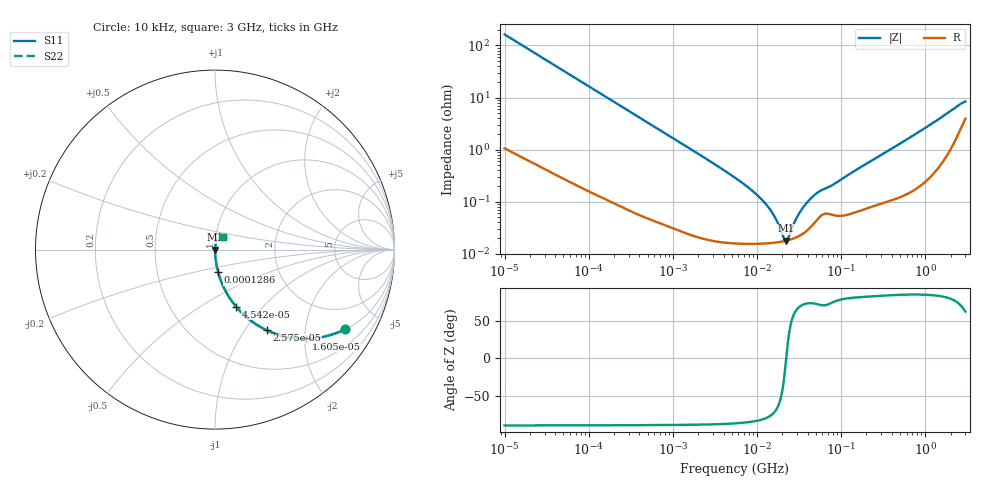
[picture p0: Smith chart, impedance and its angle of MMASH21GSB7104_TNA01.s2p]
! MMASH21GSB7104_TNA01  S-PARAMETER MODEL  ( Standard Model )
! Model Generated by TAIYO YUDEN Corporation (http://www.ty-top.com)
! Version 1.0
! TAIYO YUDEN Control No. 220601
! Copyright(c) 2013 TAIYO YUDEN CO.,LTD. All Rights Reserved.
! Product Description (link to TY-COMPAS)
! https://ds.yuden.co.jp/TYCOMPAS/or/detail?pn=MMASH21GSB7104KTNA01&u=M
! Products Name : Multilayer Ceramic Capacitors
! Characteristics :
!  Capacitance : 0.1 [uF] , Rated Voltage : 100 [V] , TCC : X7R
!  Case Size : 2.0 x 1.25 / 0.079 x 0.049 [mm/inch] , Thickness : 1.25 / 0.049 [mm/inch]
!  (Conditions: Temperature = 25 [degC] , DC Bias Voltage = 0 [V])
! External Node Assignments :
!  1  o---| |---o  2
! GND o---------o GND
! Frequency Range : 10kHz  -  3GHz  [ 401 STEP ]
# MHZ S RI R 50
! Freq[MHz].  S11 Real  S11 Imag  S21 Real  S21 Imag  S12 Real  S12 Imag  S22 Real  S22 Imag
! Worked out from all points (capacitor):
!   401 points, 10 kHz to 3 GHz, reference 50 ohm
!   read as one part in series: C = 97.7 nF near 10.65 kHz
!   lowest |Z| = 17.9 mohm at 21.93 MHz (marker M1)
!   series resonance near 22.24 MHz, so ESL is about 520 pH
!   S11 on the Smith chart (normalised r, x): 10 kHz: 1.02, -3.26; 16.05 kHz: 1.01, -2.03; 25.75 kHz: 1.01, -1.27; 45.42 kHz: 1.01, -0.72; 128.6 kHz: 1.00, -0.26; 3 GHz: 1.08, +0.15
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0.01  0.7247 -0.4434  0.2753 0.4434  0.2753 0.4434  0.7247 -0.4434
0.016047  0.5081 -0.4964  0.4919 0.4964  0.4919 0.4964  0.5081 -0.4964
0.02575  0.2886 -0.4494  0.7114 0.4494  0.7114 0.4494  0.2886 -0.4494
0.045421  0.1172 -0.3176  0.8828 0.3176  0.8828 0.3176  0.1172 -0.3176
0.082683  0.0397 -0.1906  0.9603 0.1906  0.9603 0.1906  0.0397 -0.1906
0.128563  0.0174 -0.1258  0.9826 0.1258  0.9826 0.1258  0.0174 -0.1258
0.683653  0.000984 -0.0243  0.999 0.0243  0.999 0.0243  0.000984 -0.0243
5.477226  0.000166 -0.00289  0.9998 0.00289  0.9998 0.00289  0.000166 -0.00289
9.070798  0.000157 -0.00155  0.9998 0.00155  0.9998 0.00155  0.000157 -0.00155
12.83117  0.000159 -0.000877  0.9998 0.000877  0.9998 0.000877  0.000159 -0.000877
15.99985  0.000163 -0.000509  0.9998 0.000509  0.9998 0.000509  0.000163 -0.000509
20.5901  0.000174 -0.000117  0.9998 0.000117  0.9998 0.000117  0.000174 -0.000117
21.93027  0.000178 -2.12e-05  0.9998 2.12e-05  0.9998 2.12e-05  0.000178 -2.12e-05
23.35767  0.000182 7.5e-05  0.9998 -7.5e-05  0.9998 -7.5e-05  0.000182 7.5e-05
28.22191  0.000202 0.000368  0.9998 -0.000368  0.9998 -0.000368  0.000202 0.000368
32.0153  0.000223 0.000571  0.9998 -0.000571  0.9998 -0.000571  0.000223 0.000571
45.28751  0.000352 0.00118  0.9996 -0.00118  0.9996 -0.00118  0.000352 0.00118
54.71863  0.0005 0.00149  0.9995 -0.00149  0.9995 -0.00149  0.0005 0.00149
79.88199  0.000561 0.00204  0.9994 -0.00204  0.9994 -0.00204  0.000561 0.00204
374.4521  0.00112 0.00975  0.9989 -0.00975  0.9989 -0.00975  0.00112 0.00975
2482.93  0.0243 0.0651  0.9757 -0.0651  0.9757 -0.0651  0.0243 0.0651
3000  0.0426 0.0686  0.9574 -0.0686  0.9574 -0.0686  0.0426 0.0686
